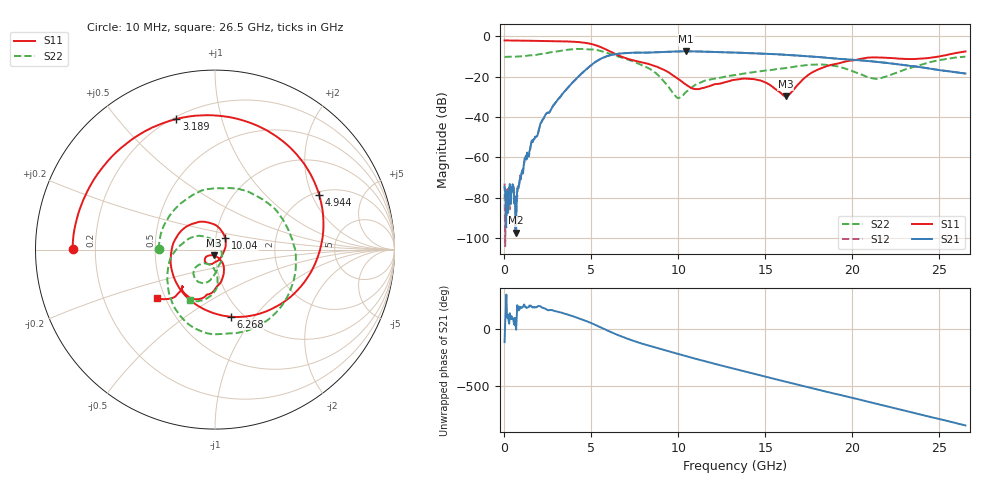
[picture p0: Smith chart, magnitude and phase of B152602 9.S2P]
!  2-Port S-parameters saved by WinCal
! VAR MeasName=S-Parameters (CALIBRATED_DATA) read from VNA (N5242A)
! VAR MeasDate=2016-1-5 16:26:47
! VAR NAME=B152602 9
! VAR FILENAME=B152602 9.S2P
! VAR DATE=2016-1-5 16:26:47
! VAR PHYS_PORTS=1,2
# Hz S DB R 50
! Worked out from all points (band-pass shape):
!   801 points, 10 MHz to 26.5 GHz, reference 50 ohm
!   highest |S21| = -7.37 dB at 10.44 GHz (marker M1); lowest = -97.2 dB at 639.1 MHz (marker M2)
!   |S21| within 3 dB of the highest: 5.722 GHz to 18.26 GHz (12.54 GHz wide, 105 % of centre)
!   lowest |S11| = -29.7 dB at 16.17 GHz (marker M3), VSWR 1.07, Z = 49.1 - j3.11 ohm
!   |S11| at or under -10 dB: 6.712 GHz to 24.95 GHz (18.24 GHz wide, 115 % of centre)
!   |S22| runs from -30.6 to -6.2 dB; largest |S21 - S12| = 0.0026
!   S11 on the Smith chart (normalised r, x): 10 MHz: 0.12, +0.00; 3.189 GHz: 0.21, +0.73; 4.944 GHz: 2.12, +2.27; 6.268 GHz: 0.88, -0.77; 10.04 GHz: 1.11, +0.14; 26.5 GHz: 0.45, -0.30
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1e7  -2.01 179.7  -74.70 -114.8  -72.98 1.5  -10.16 179.5
6.391375e8  -2.06 166.8  -97.24 49.6  -79.22 133.3  -10.03 144.2
1.632512e9  -2.19 146.2  -52.32 -172.0  -52.13 -171.3  -9.34 89.0
2.294762e9  -2.27 130.9  -39.88 -179.2  -39.85 -179.1  -8.47 53.2
3.1888e9  -2.39 106.5  -30.19 146.6  -30.21 146.5  -7.19 5.5
4.447075e9  -2.97 56.5  -18.33 84.8  -18.35 84.8  -6.22 -59.8
4.943762e9  -3.67 27.7  -14.58 55.1  -14.58 55.2  -6.51 -82.9
5.506675e9  -5.19 -12.8  -11.23 16.0  -11.23 16.0  -7.13 -109.8
6.268262e9  -8.32 -76.8  -8.97 -36.9  -8.96 -36.9  -9.22 -138.4
7.261638e9  -11.51 -155.7  -8.12 -95.4  -8.12 -95.5  -11.90 -168.6
8.851038e9  -15.35 114.5  -7.78 -169.6  -7.79 -169.7  -19.35 135.2
1.004309e10  -21.34 47.3  -7.42 138.9  -7.41 139.0  -30.53 26.1
1.044044e10  -23.94 19.7  -7.37 121.7  -7.37 121.8  -27.52 -25.0
1.16656e10  -24.96 -59.5  -7.59 71.0  -7.58 71.1  -21.61 -70.2
1.3255e10  -21.49 -106.3  -8.02 9.0  -8.01 8.9  -19.11 -83.9
1.471195e10  -21.83 -135.1  -8.52 -46.8  -8.50 -46.8  -17.31 -90.5
1.61689e10  -29.71 -104.6  -9.16 -102.1  -9.15 -102.3  -15.67 -97.3
1.769208e10  -17.83 -66.9  -9.99 -159.8  -9.97 -159.6  -14.00 -111.1
1.997684e10  -11.94 -99.4  -11.58 116.5  -11.56 116.4  -17.10 -137.4
2.209604e10  -10.63 -127.2  -13.29 37.1  -13.24 36.8  -19.43 -93.1
2.43808e10  -10.71 -130.0  -15.87 -47.9  -15.84 -48.1  -12.95 -89.0
2.65e10  -7.47 -140.0  -18.41 -126.4  -18.38 -126.8  -10.05 -115.8
